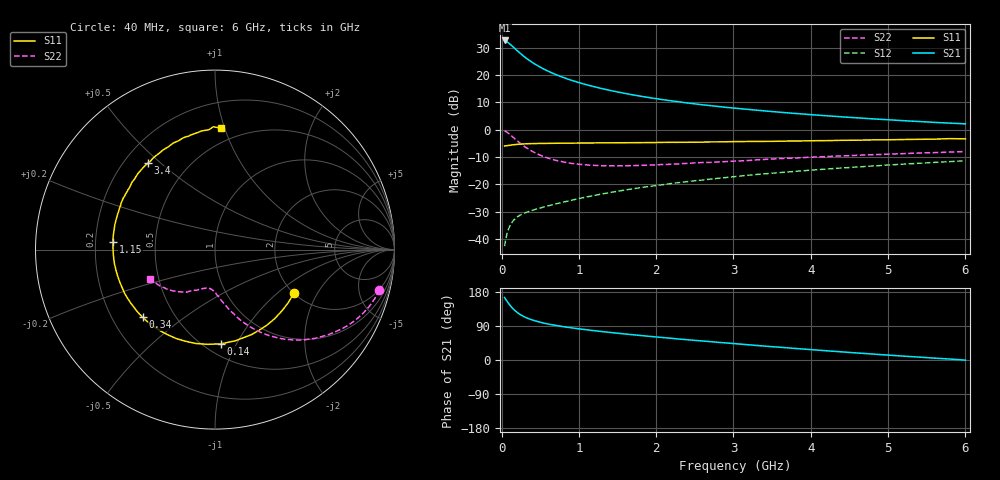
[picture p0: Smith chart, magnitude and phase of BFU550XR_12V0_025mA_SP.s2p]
! Filename:  P:\Prog\Test\Noise\ATS_data\Testdata_Net\03 Spar\BFU550XR_APG2013_45_C05_12p0V_025mA_SP_CM01_D.s2p
! Date/Time: Tue 06/Aug/2013 14:38:19
! BFU550XR_APG2013_45_C05_12p0V_25to35mA_SP_CM01_Bias1_R.s2p
! MDIF S-parameter v. bias file
! BFU550XR_APG2013_45_C05_12p0V_25to35mA_SP_CM01
! Date/time Mon Aug 05 17:40:26 2013
! bias mode 1
! bias variable = I_out
! VAR bias_var= 1
! VAR V_out= 12.0010
! VAR I_out= 25.0000
! VAR V_in= 0.7730
! VAR I_in= 0.2438
! Device data file deembeded for feedlines and parallel
! Original file: \03 Spar\BFU550XR_APG2013_45_C05_12p0V_025mA_SP_CM01_R.s2p
! Feed-files: PR006V01_02082013_Feed1.s2p, PR006V01_02082013_Feed2.s2p
! Parallel-file: PR006V01_02082013_Par.s2p
# MHz S MA R 50
!  Freq-MHz  S11-mag  S11-arg  S21-mag  S21-arg  S12-mag  S12-arg  S22-mag  S22-arg
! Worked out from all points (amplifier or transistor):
!   98 points, 40 MHz to 6 GHz, reference 50 ohm
!   highest |S21| = 32.6 dB at 40 MHz (marker M1)
!   |S21| within 3 dB of that: start of sweep to 174.3 MHz
!   unconditionally stable (mu >= 1): 1.508 GHz to 3.265 GHz; 3.485 GHz to 3.504 GHz
!   at 300 MHz: K = 0.47, MSG = 28.5 dB, |S12| = -30.5 dB
!   at 1.6 GHz: K = 1.01, MAG = 17.1 dB, |S12| = -22.1 dB
!   at 6 GHz: K = 0.88, MSG = 6.8 dB, |S12| = -11.4 dB
!   S11 on the Smith chart (normalised r, x): 40 MHz: 2.00, -1.30; 140 MHz: 0.60, -0.87; 340 MHz: 0.33, -0.36; 1.15 GHz: 0.27, +0.04; 3.4 GHz: 0.30, +0.46; 6 GHz: 0.39, +0.97
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40  0.5025 -29.0  42.74 165.0  0.007384 76.8  0.9435 -13.8
50  0.5041 -35.9  41.85 161.2  0.009017 75.0  0.9307 -17.2
70  0.5086 -49.3  40.4 155.6  0.01223 71.0  0.8965 -23.5
90  0.5123 -61.4  38.51 149.6  0.01501 67.1  0.8553 -29.4
120  0.5204 -77.3  35.61 141.8  0.01855 62.2  0.7889 -37.0
140  0.5261 -86.3  33.6 137.3  0.0205 59.5  0.7455 -41.5
180  0.5337 -101.5  29.76 129.4  0.02375 55.3  0.6646 -49.2
220  0.5404 -113.5  26.51 123.0  0.02622 52.6  0.5953 -55.3
280  0.5472 -127.0  22.45 115.6  0.02904 50.3  0.5115 -62.3
340  0.5515 -136.9  19.31 110.0  0.03137 49.3  0.4486 -67.5
440  0.5561 -148.8  15.55 103.0  0.03488 49.5  0.3728 -73.7
600  0.5607 -161.4  11.78 95.1  0.04023 51.2  0.302 -80.8
800  0.5657 -171.9  8.991 88.0  0.04728 53.7  0.2569 -86.8
1050  0.5683 178.7  6.919 81.0  0.05665 56.2  0.2292 -92.2
1150  0.5699 175.5  6.335 78.5  0.06056 56.8  0.2233 -94.3
1550  0.5751 164.7  4.735 69.7  0.07666 58.0  0.2175 -100.9
2050  0.5835 153.7  3.592 59.9  0.09699 57.6  0.2292 -107.8
3100  0.6048 133.2  2.409 41.7  0.1421 53.5  0.2682 -120.6
3400  0.6092 127.7  2.2 36.7  0.1554 51.4  0.2853 -123.8
4100  0.6277 116.0  1.834 25.9  0.1855 46.9  0.3167 -132.6
5200  0.659 98.6  1.456 10.2  0.2338 38.6  0.3639 -145.8
6000  0.6777 87.4  1.274 -0.4  0.2689 31.7  0.3976 -155.8
